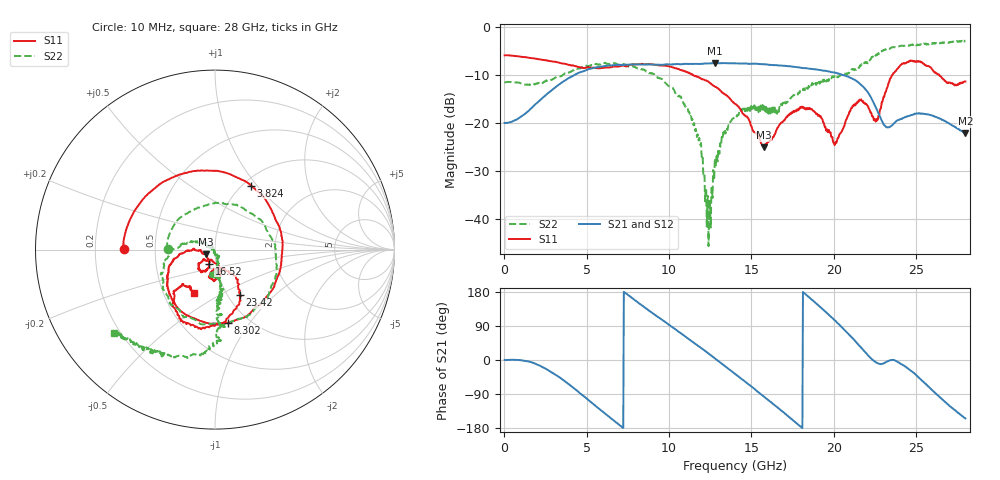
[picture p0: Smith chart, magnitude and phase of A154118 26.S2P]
!  2-Port S-parameters saved by WinCal
! VAR MeasName=S-Parameters (CALIBRATED_DATA) read from VNA (N5230A)
! VAR MeasDate=2015-9-10 14:36:21
! VAR NAME=A154118 26
! VAR FILENAME=A154118 26.S2P
! VAR DATE=2015-9-10 14:36:21
! VAR PHYS_PORTS=1,2
# Hz S DB R 50
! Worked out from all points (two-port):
!   801 points, 10 MHz to 28 GHz, reference 50 ohm
!   highest |S21| = -7.44 dB at 12.78 GHz (marker M1); lowest = -22.1 dB at 28 GHz (marker M2)
!   |S21| within 3 dB of the highest: 3.99 GHz to 20.95 GHz (16.95 GHz wide, 136 % of centre)
!   lowest |S11| = -25.0 dB at 15.75 GHz (marker M3), VSWR 1.12, Z = 45.3 - j2.43 ohm
!   |S11| at or under -10 dB: 11.46 GHz to 23.55 GHz (12.09 GHz wide, 69 % of centre); 26.42 GHz to end of sweep
!   |S22| runs from -45.8 to -2.7 dB; largest |S21 - S12| = 0.0076
!   S11 on the Smith chart (normalised r, x): 10 MHz: 0.32, +0.00; 3.824 GHz: 1.09, +0.93; 8.302 GHz: 0.81, -0.79; 16.52 GHz: 0.92, -0.14; 23.42 GHz: 1.14, -0.63; 28 GHz: 0.71, -0.37
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1e7  -5.86 179.6  -19.99 0.1  -20.00 0.0  -11.63 179.9
2.074262e9  -6.65 118.8  -15.50 -13.7  -15.50 -13.4  -11.71 86.3
3.823638e9  -7.76 60.6  -10.77 -61.2  -10.75 -61.1  -9.50 1.8
4.698325e9  -8.43 29.5  -9.29 -91.4  -9.28 -91.6  -8.38 -36.1
6.097825e9  -8.41 -16.6  -8.10 -140.8  -8.08 -140.6  -7.41 -83.4
8.302038e9  -7.65 -80.0  -7.77 145.5  -7.74 145.5  -8.80 -141.3
9.351662e9  -7.95 -105.4  -7.83 112.6  -7.77 112.5  -10.53 -164.3
1.14859e10  -10.05 -147.4  -7.63 45.9  -7.58 45.4  -20.49 154.5
1.190575e10  -10.62 -153.2  -7.65 32.9  -7.59 32.3  -24.53 143.6
1.239558e10  -11.40 -160.4  -7.53 17.2  -7.47 16.5  -45.76 -158.6
1.278044e10  -12.38 -165.1  -7.44 4.7  -7.41 4.0  -27.39 -78.0
1.4005e10  -15.97 -177.6  -7.53 -36.4  -7.52 -37.0  -18.77 -86.8
1.575438e10  -25.05 -151.4  -7.73 -96.5  -7.73 -96.8  -17.48 -97.5
1.65241e10  -21.48 -113.2  -7.90 -123.0  -7.86 -123.4  -17.19 -83.1
1.869332e10  -17.14 -131.5  -8.69 158.6  -8.75 158.1  -11.64 -82.1
2.009282e10  -24.27 -110.8  -9.47 103.7  -9.53 103.1  -10.40 -85.6
2.152731e10  -15.50 -90.9  -11.59 38.9  -11.56 38.2  -8.53 -86.7
2.261192e10  -19.15 -74.7  -17.11 -7.1  -17.10 -7.7  -5.62 -88.8
2.334666e10  -11.51 -58.6  -20.91 -2.2  -20.92 -2.6  -4.52 -100.1
2.341664e10  -10.78 -61.3  -20.82 -1.0  -20.82 -1.2  -4.39 -102.7
2.572581e10  -8.08 -127.4  -18.16 -69.2  -18.20 -69.5  -3.52 -122.7
2.8e10  -11.31 -116.1  -22.15 -154.2  -22.18 -154.5  -2.74 -140.2
